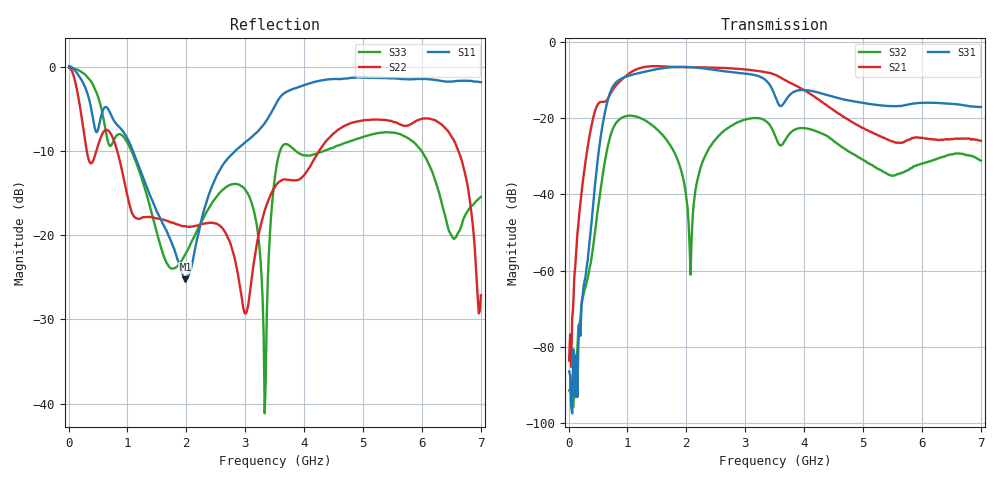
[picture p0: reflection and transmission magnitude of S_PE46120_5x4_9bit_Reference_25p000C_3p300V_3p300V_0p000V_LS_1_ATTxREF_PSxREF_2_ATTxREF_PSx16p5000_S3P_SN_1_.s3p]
! Device ID: PE46120_5x4_9bit_Reference
! Device ID: PE46120_5x4_9bit_Reference
! File Path: z:\PE46120_5x4_9bit_Reference\MPAC_Yi\new_12port\25p000C\3p300\LS_1_ATTxREF_PSxREF_2_ATTxREF_PSx16p5000\PE46120_5x4_9bit_Reference_25p000C_3p300V_3p300V_0p000V_LS_1_ATTxREF_PSxREF_2_ATTxREF_PSx16p5000_S3P_SN_1_.s3p
! Serial: 1
! Lot:
! Temp: 25.000C
! VDD: 3.300
! VSS: 0.000
! Control_Hi: 3.300
! Control_Lo: 0.000
! Logic State: LS_1_ATTxREF_PSxREF_2_ATTxREF_PSx16p5000
! Port 1: RFin
! Port 2: RFout1
! Port 3: RFout2
! ThroughPath:1-3
! IDD: -0.000538665
! ISS: 0
! Comment:
#  Hz  S  RI  R  50
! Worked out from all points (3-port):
!   401 points, 10 MHz to 7 GHz, reference 50 ohm
!   strongest paths, dB at 10 MHz, 1.758 GHz, 3.505 GHz, 5.253 GHz, 7 GHz:
!     S31: -86.4, -6.7, -14.2, -16.6, -17.1
!     S21: -83.6, -6.6, -8.7, -24.5, -26.0
!     S32: -91.4, -27.9, -24.6, -33.3, -31.2
!   lowest |S11| = -25.3 dB at 1.985 GHz (marker M1), VSWR 1.12, Z = 54.1 + j3.9 ohm
!   |S11| at or under -10 dB: 1.092 GHz to 2.831 GHz (1.739 GHz wide, 88.6 % of centre)
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1e7  1.001 -0.1151  2.74e-05 0.000107  -9.99e-05 5.32e-05
     3.24e-05 -5.78e-05  0.9872 -0.0962  -2.74e-05 -2.82e-05
     3.66e-05 3.07e-05  2.65e-05 -4.42e-06  0.983 -0.0312
2.5465e8  -0.5334 -0.5873  -0.0162 -0.00574  0.000258 -0.000492
          -0.0163 -0.00593  -0.3264 -0.2675  -0.000436 0.000208
          0.000224 -0.000562  -0.00044 0.000207  0.6463 -0.6444
4.81825e8  -0.3987 -0.0883  -0.0448 0.134  0.0117 -0.0194
           -0.0455 0.1357  0.1908 0.2623  0.00102 0.00498
           0.0119 -0.0196  0.00106 0.00508  0.0119 -0.6925
9.71125e8  -0.2764 0.275  0.3366 -0.0938  0.1453 0.3099
           0.3409 -0.0949  -0.058 -0.1811  0.0263 0.101
           0.1472 0.314  0.0267 0.1023  -0.279 -0.2396
1.984675e9  0.0411 0.0359  -0.3705 0.2676  -0.3984 -0.2316
            -0.3749 0.2711  -0.0911 0.0665  0.00403 0.0105
            -0.404 -0.2342  0.00409 0.0103  -0.0609 0.0474
2.98075e9  -0.1679 -0.3083  0.4128 -0.1165  0.2125 0.3127
           0.4181 -0.1189  -0.0029 -0.0349  0.0894 0.0273
           0.2157 0.3164  0.0904 0.0277  0.1792 0.0623
3.33025e9  -0.2808 -0.3672  0.1056 -0.3819  0.3161 -0.0256
           0.1068 -0.3871  -0.0517 0.1302  0.0176 -0.0905
           0.3203 -0.0262  0.0177 -0.0915  0.00863 -0.00146
3.505e9  -0.3944 -0.4375  -0.1035 -0.3495  0.1605 -0.1066
         -0.1049 -0.3541  0.0589 0.1846  -0.0361 -0.0462
         0.1625 -0.1083  -0.0366 -0.0465  0.1009 0.1987
6.248575e9  -0.3799 0.7416  0.0397 -0.0324  0.0522 0.1464
            0.0403 -0.0329  0.466 -0.0924  -0.0278 0.00775
            0.053 0.1483  -0.0278 0.0082  -0.0806 -0.182
7e9  -0.1093 0.8022  -0.028 -0.0407  0.137 -0.0055
     -0.0289 -0.0411  -0.0398 0.0186  0.0267 -0.0027
     0.1395 -0.00614  0.0275 -0.00278  0.0502 0.1609
